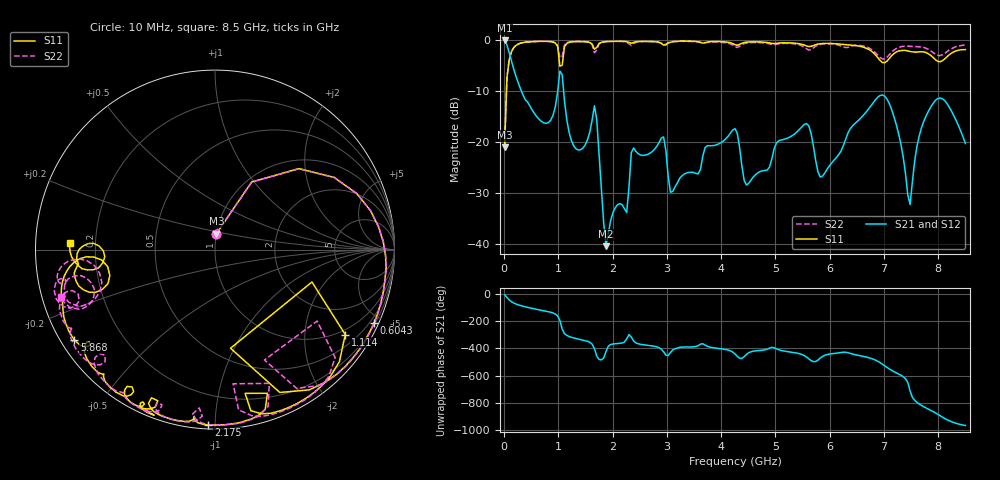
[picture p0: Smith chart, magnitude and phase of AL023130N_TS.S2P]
!AVX Corporation
!PN: AL023130N_TS
!DESCRIPTION: AIR CORE INDUCTOR, 130nH, 11 turns
!Agilent Technologies,E5071C,MY46102230,A.09.54
!Date: Mon Sep 03 16:44:42 2012
!Data & Calibration Information:
!Freq	S11:SOLT2(ON)	S21:SOLT2(ON)	S12:SOLT2(ON)	S22:SOLT2(ON)
# Hz S dB R 50
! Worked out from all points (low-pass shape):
!   201 points, 10 MHz to 8.5 GHz, reference 50 ohm
!   highest |S21| = -0.03 dB at 10 MHz (marker M1); lowest = -40.4 dB at 1.878 GHz (marker M2)
!   |S21| within 3 dB of the highest: start of sweep to 109.9 MHz
!   lowest |S11| = -21.0 dB at 10 MHz (marker M3), VSWR 1.20, Z = 50 + j8.93 ohm
!   |S11| at or under -10 dB: start of sweep to 44.27 MHz
!   |S22| runs from -20.9 to -0.2 dB; largest |S21 - S12| = 0.0051
!   S11 on the Smith chart (normalised r, x): 10 MHz: 1.00, +0.18; 604.3 MHz: 0.26, -4.52; 1.114 GHz: 0.83, -3.16; 2.175 GHz: 0.02, -0.96; 5.868 GHz: 0.04, -0.29; 8.5 GHz: 0.10, +0.02
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1e7  -21.02 84.9  -0.03 -5.7  -0.03 -6.0  -20.92 85.2
5.245e7  -7.37 61.6  -0.90 -28.2  -0.88 -28.4  -7.36 61.3
1.3735e8  -2.20 31.2  -4.11 -58.5  -4.10 -58.6  -2.18 31.1
6.043e8  -0.21 -24.9  -15.00 -113.9  -14.99 -114.1  -0.21 -25.1
1.0288e9  -5.10 -81.1  -6.04 164.3  -6.03 164.2  -3.43 -65.9
1.07125e9  -4.89 -18.5  -6.79 100.0  -6.79 100.0  -3.17 -35.0
1.1137e9  -1.25 -33.1  -11.96 68.1  -11.96 68.0  -0.92 -41.9
1.4533e9  -0.26 -66.1  -21.15 20.4  -21.15 20.2  -0.23 -68.9
1.66555e9  -1.74 -78.2  -12.85 -42.9  -12.84 -42.9  -2.45 -82.3
1.8778e9  -0.27 -80.2  -40.42 -63.9  -40.35 -63.1  -0.24 -80.2
2.17495e9  -0.20 -92.2  -32.26 -1.2  -32.28 -1.2  -0.22 -92.5
2.3872e9  -0.41 -97.3  -21.14 13.3  -21.12 13.3  -0.62 -94.4
2.85415e9  -0.41 -112.0  -20.11 -34.9  -20.09 -34.9  -0.37 -109.6
3.0664e9  -0.37 -112.2  -29.84 -70.6  -29.86 -70.6  -0.32 -110.3
4.255e9  -0.86 -122.7  -17.36 -80.8  -17.37 -80.8  -1.25 -138.0
4.46725e9  -0.34 -122.0  -28.42 -83.6  -28.46 -83.6  -0.54 -137.9
5.6983e9  -1.02 -142.7  -20.69 -137.4  -20.69 -137.5  -1.51 -157.9
5.8681e9  -0.63 -147.3  -26.67 -99.3  -26.68 -99.0  -0.72 -161.6
7.09915e9  -3.54 -160.6  -12.45 168.6  -12.45 168.5  -2.82 -157.6
7.4812e9  -2.20 -172.9  -32.25 7.2  -32.27 7.7  -1.18 -163.9
7.94815e9  -3.81 178.3  -11.79 -152.7  -11.80 -152.7  -2.72 -167.3
8.5e9  -1.82 177.3  -20.27 114.8  -20.30 114.9  -0.94 -162.8
